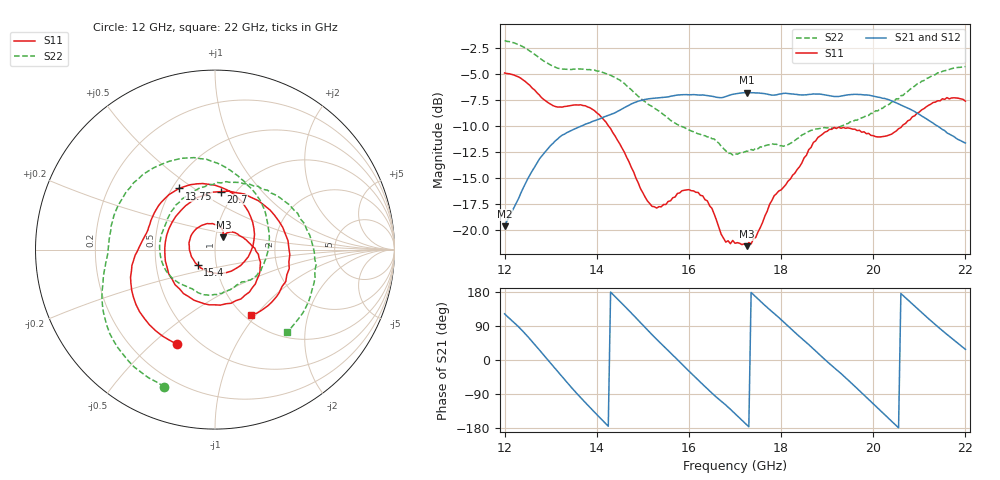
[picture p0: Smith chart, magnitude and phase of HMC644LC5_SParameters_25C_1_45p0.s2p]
!Analog Devices Inc..
!GaAs MMIC 5-BIT DIGITAL PHASE SHIFTER, 15 -8.5 GHz
!Filename: HMC644LC5_sparm_25C_1_0.s2p
!  :25C = 25degC
!  :_1_ = Sn1
!  :_45p0  = 45deg
!Device type:
!2 Port Calibration to sma connectors
!Phase Shifter:  0.000
!	50 Ohm System, Control Voltage = 0/-3V
!Freq	S11	S11	S21	S21	S12	S12	S22	S22
! GHz	Mag dB	Degrees	Mag dB	Degrees	Mag dB	Degrees	Mag dB	Degrees
# GHZ S DB R 50.0
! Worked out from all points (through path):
!   201 points, 12 GHz to 22 GHz, reference 50 ohm
!   highest |S21| = -6.80 dB at 17.25 GHz (marker M1); lowest = -19.6 dB at 12 GHz (marker M2)
!   lowest |S11| = -21.6 dB at 17.25 GHz (marker M3), VSWR 1.18, Z = 54.4 + j7.55 ohm
!   |S11| at or under -10 dB: 14.25 GHz to 20.63 GHz (6.376 GHz wide, 36.6 % of centre)
!   |S22| runs from -12.8 to -1.8 dB; largest |S21 - S12| = 0.0027
!   S11 on the Smith chart (normalised r, x): 12 GHz: 0.39, -0.61; 13.75 GHz: 0.54, +0.44; 15.4 GHz: 0.81, -0.14; 20.7 GHz: 0.86, +0.62; 22 GHz: 1.07, -0.94
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12  -4.91 -111.7  -19.65 121.9  -19.68 121.6  -1.78 -110.3
12.45  -5.73 -153.8  -15.56 69.0  -15.54 69.0  -2.50 -141.5
13.05  -8.05 168.4  -11.68 -15.9  -11.64 -15.8  -4.25 -173.1
13.7  -8.04 125.3  -9.95 -105.7  -9.94 -105.6  -4.54 155.7
13.75  -8.06 120.5  -9.84 -112.2  -9.86 -112.1  -4.57 153.0
14.5  -11.73 35.8  -8.49 155.1  -8.51 155.1  -5.59 102.8
14.95  -16.04 -41.4  -7.57 98.4  -7.55 98.5  -7.32 72.8
15.35  -17.77 -127.0  -7.30 48.6  -7.28 48.7  -8.58 47.6
15.4  -17.78 -137.6  -7.29 42.6  -7.28 42.5  -8.74 44.5
15.85  -16.24 151.2  -7.00 -11.2  -6.98 -11.3  -10.07 16.2
16.3  -16.73 95.7  -7.02 -64.4  -7.02 -64.2  -10.93 -14.0
17  -21.29 60.5  -6.92 -141.5  -6.91 -141.3  -12.67 -56.7
17.25  -21.57 55.7  -6.80 -170.4  -6.79 -170.4  -12.43 -69.2
17.6  -19.27 55.3  -6.88 149.7  -6.86 149.6  -12.05 -90.2
18.05  -15.91 27.9  -6.87 100.9  -6.87 100.9  -11.96 -120.1
18.7  -11.60 -15.4  -6.92 29.6  -6.93 29.5  -10.38 -165.5
19.15  -10.15 -62.1  -7.17 -20.1  -7.16 -20.0  -10.21 157.4
19.65  -10.45 -119.8  -6.97 -75.1  -6.96 -75.0  -9.45 119.5
20.35  -10.87 140.0  -7.50 -156.1  -7.51 -155.9  -7.91 65.7
20.7  -9.77 84.2  -8.18 164.1  -8.19 164.3  -6.80 41.3
21.3  -7.75 7.0  -9.73 98.4  -9.75 98.5  -5.14 -1.5
22  -7.62 -61.1  -11.65 28.1  -11.73 28.2  -4.29 -48.8
